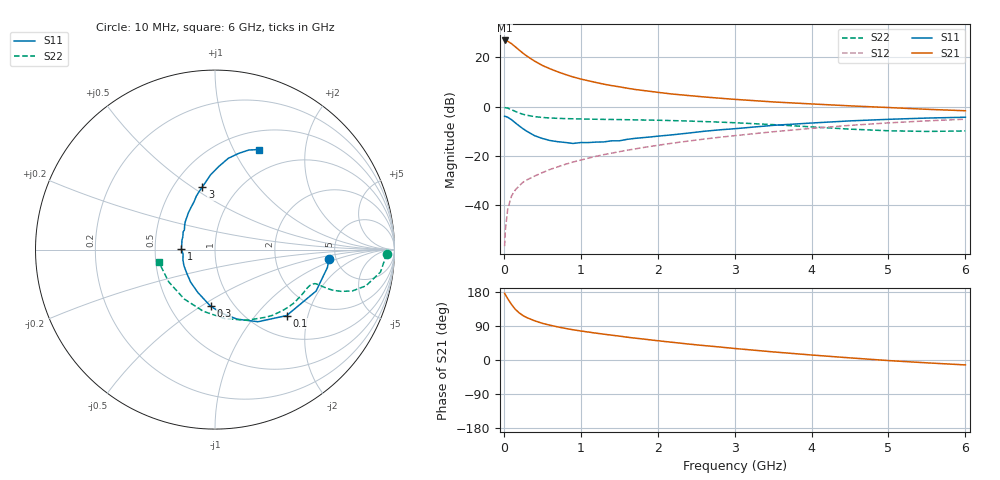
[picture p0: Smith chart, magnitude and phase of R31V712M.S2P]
! SIEMENS Small Signal Semiconductors
! BFR181
! Si NPN RF Bipolar Junction Transistor in SOT23
! VCE = 1.75 V  IC = 12 mA
! Common Emitter S-Parameters:  May  1996
# GHz  S  MA  R  50
!  f  S11  S21  S12  S22
! GHz  MAG  ANG  MAG  ANG  MAG  ANG  MAG  ANG
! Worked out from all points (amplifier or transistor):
!   36 points, 10 MHz to 6 GHz, reference 50 ohm
!   highest |S21| = 26.8 dB at 10 MHz (marker M1)
!   |S21| within 3 dB of that: start of sweep to 165.6 MHz
!   unconditionally stable (mu >= 1): 464.7 MHz to 2.912 GHz
!   at 250 MHz: K = 0.74, MSG = 26.1 dB, |S12| = -30.6 dB
!   at 1.4 GHz: K = 1.15, MAG = 11.4 dB, |S12| = -18.9 dB
!   at 6 GHz: K = 0.91, MSG = 1.7 dB, |S12| = -5.1 dB
!   S11 on the Smith chart (normalised r, x): 10 MHz: 4.35, -0.78; 100 MHz: 1.42, -1.48; 300 MHz: 0.78, -0.55; 1 GHz: 0.68, +0.01; 3 GHz: 0.69, +0.55; 6 GHz: 0.72, +1.27
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0.01  0.6358 -4.8  21.79 176.2  0.0015 100.4  0.9569 -1.4
0.02  0.6346 -8.9  21.6 172.4  0.0032 83.7  0.9486 -3.1
0.05  0.6088 -22.3  21.01 161.9  0.0084 80.7  0.9307 -7.7
0.1  0.5428 -42.6  18.74 146.4  0.0156 72.3  0.8649 -13.5
0.15  0.4679 -59.2  16.16 133.6  0.0207 67.7  0.7982 -16.8
0.2  0.4065 -72.4  13.91 124.3  0.025 67.1  0.7408 -18.3
0.25  0.3558 -84.0  12 117.2  0.0295 65.8  0.6978 -19.0
0.3  0.3165 -94.4  10.52 111.7  0.0329 66.4  0.6684 -19.1
0.4  0.2578 -111.6  8.319 103.5  0.0393 67.1  0.6279 -18.9
0.5  0.2267 -126.8  6.809 96.8  0.0461 68.3  0.6026 -18.7
0.6  0.206 -139.3  5.823 91.8  0.0534 69.0  0.588 -18.8
0.7  0.1951 -152.3  5.063 87.4  0.0603 69.8  0.5788 -19.3
0.9  0.1797 -171.8  3.975 79.8  0.0756 70.8  0.5663 -20.5
1  0.1872 178.4  3.615 76.6  0.0828 71.2  0.5616 -21.4
1.1  0.1873 171.2  3.327 73.7  0.0908 71.4  0.5574 -22.4
1.6  0.2172 141.0  2.361 60.3  0.1306 70.2  0.543 -28.5
2.2  0.2695 119.9  1.788 46.5  0.1827 67.1  0.5203 -37.7
3  0.3568 101.3  1.402 30.4  0.2583 60.7  0.4717 -53.0
3.5  0.4173 93.4  1.243 21.4  0.3098 55.7  0.4316 -65.7
4.5  0.5141 81.7  1.035 5.6  0.4171 43.4  0.3499 -100.7
5.5  0.5863 71.2  0.882 -7.5  0.5147 29.0  0.3144 -145.1
6  0.6094 66.1  0.824 -13.0  0.5561 21.3  0.3216 -168.1
